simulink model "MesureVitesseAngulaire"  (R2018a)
settings: Solver=FixedStepAuto  StartTime=0.0  StopTime=inf  RelTol=1e-3  EnableMultiTasking=on
undefined symbols (not defined in the file): hex2dec
libraries: arduinolib x2, dspindex x1

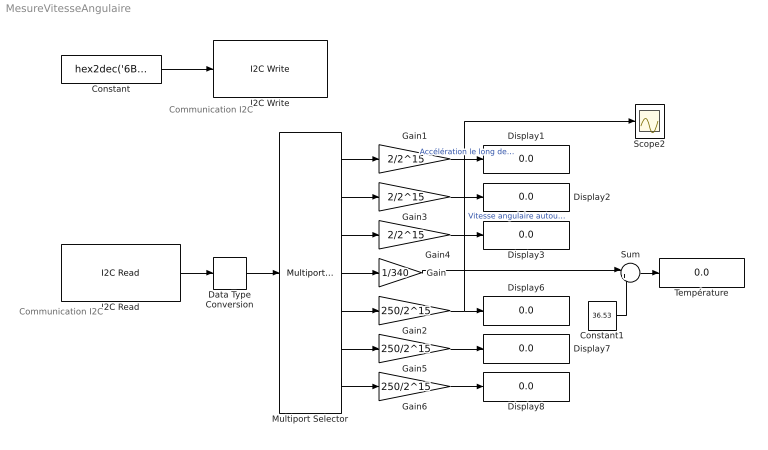
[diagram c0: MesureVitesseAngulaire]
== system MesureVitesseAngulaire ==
  note: Communication I2C
  note: Communication I2C
  Constant : Constant  Value=hex2dec('6B00')  OutDataTypeStr=uint16  SampleTime=0.01
  Constant1 : Constant  Value=36.53
  Data Type Conversion : DataTypeConversion  OutDataTypeStr=int16
  Display{1..3,6..8} (6 alike) : Display
  Gain : Gain  Gain=1/340
  Gain1 : Gain  Gain=2/2^15
  Gain2 : Gain  Gain=250/2^15
  Gain3 : Gain  Gain=2/2^15
  Gain4 : Gain  Gain=2/2^15
  Gain5 : Gain  Gain=250/2^15
  Gain6 : Gain  Gain=250/2^15
  I2C Read : arduinolib/I2C Read  SlaveAddress_=hex2dec( '68' )  RegisterAddressEnable=on  RegisterAddress_=hex2dec( '3B' )  Datatype=uint16  ByteOrder=Big Endian  Datalength_=7  SampleTime_=-1  blockPlatform=arduino
  I2C Write : arduinolib/I2C Write  SlaveAddress_=hex2dec( '68' )  RegisterAddressEnable=off  RegisterAddress_=hex2dec( '00' )  Datatype=uint16  ByteOrder=Big Endian  blockPlatform=arduino
  Multiport Selector : dspindex/Multiport Selector  rowsOrCols=Rows  idxCellArray={ 1, 2, 3, 4, 5, 6, 7 }  idxErrMode=Clip Index
  Scope2 : Scope
  Sum : Sum  Inputs=|++
  Température : Display
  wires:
  Constant/1 -> I2C Write/1
  I2C Read/1 -> Data Type Conversion/1
  Data Type Conversion/1 -> Multiport Selector/1
  Multiport Selector/1 -> Gain1/1
  Gain/1 -> Sum/1
  Constant1/1 -> Sum/2
  Sum/1 -> Température/1
  Gain2/1 -> Scope2/1, Display6/1  "Vitesse angulaire autour de l'axe X en rad/s"
  Gain3/1 -> Display2/1
  Multiport Selector/2 -> Gain3/1
  Gain4/1 -> Display3/1
  Multiport Selector/3 -> Gain4/1
  Multiport Selector/4 -> Gain/1
  Multiport Selector/5 -> Gain2/1
  Gain5/1 -> Display7/1
  Multiport Selector/6 -> Gain5/1
  Multiport Selector/7 -> Gain6/1
  Gain1/1 -> Display1/1  "Accélération le long de l'axe X"
  Gain6/1 -> Display8/1
